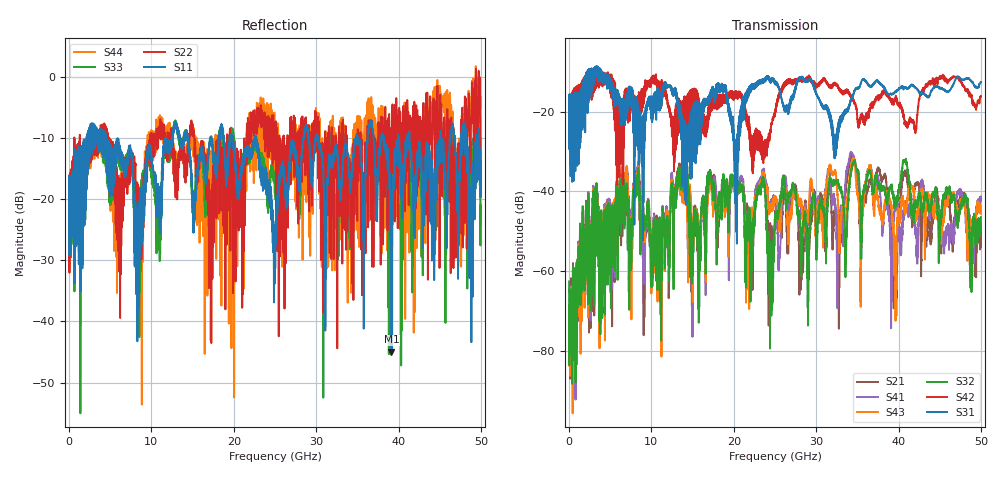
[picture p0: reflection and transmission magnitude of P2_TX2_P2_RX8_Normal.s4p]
!Keysight Technologies,N5225B,MY57041031,A.13.20.10
!Date: Friday, May 31, 2019 11:39:17
!Correction: S11(Full 4 Port(1,2,3,4))
!S12(Full 4 Port(1,2,3,4))
!S13(Full 4 Port(1,2,3,4))
!S14(Full 4 Port(1,2,3,4))
!S21(Full 4 Port(1,2,3,4))
!S22(Full 4 Port(1,2,3,4))
!S23(Full 4 Port(1,2,3,4))
!S24(Full 4 Port(1,2,3,4))
!S31(Full 4 Port(1,2,3,4))
!S32(Full 4 Port(1,2,3,4))
!S33(Full 4 Port(1,2,3,4))
!S34(Full 4 Port(1,2,3,4))
!S41(Full 4 Port(1,2,3,4))
!S42(Full 4 Port(1,2,3,4))
!S43(Full 4 Port(1,2,3,4))
!S44(Full 4 Port(1,2,3,4))
!S4P File: Measurements: <S11,S12,S13,S14>,
!<S21,S22,S23,S24>,
!<S31,S32,S33,S34>,
!<S41,S42,S43,S44>:
# Hz S  dB  R 50.0
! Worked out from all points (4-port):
!   5000 points, 10 MHz to 50 GHz, reference 50 ohm
!   strongest paths, dB at 10 MHz, 12.51 GHz, 25.01 GHz, 37.51 GHz, 50 GHz:
!     S31: -19.4, -14.8, -13.0, -12.4, -12.6
!     S42: -19.7, -21.5, -19.9, -16.3, -16.1
!     S32: -62.5, -39.7, -46.8, -38.3, -46.4
!     S43: -77.9, -38.8, -41.5, -41.8, -45.6
!     S41: -68.5, -37.1, -41.9, -36.2, -41.3
!     S21: -73.2, -37.8, -45.5, -34.1, -54.0
!   lowest |S11| = -44.9 dB at 39.13 GHz (marker M1), VSWR 1.01, Z = 49.6 + j0.422 ohm
!   |S11| at or under -10 dB: 4.481 GHz to 11.72 GHz (7.237 GHz wide, 89.4 % of centre); 22.73 GHz to 28.43 GHz (5.702 GHz wide, 22.3 % of centre); 30.26 GHz to 34.82 GHz (4.558 GHz wide, 14 % of centre)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
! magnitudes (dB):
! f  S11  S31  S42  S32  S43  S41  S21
! 10 MHz  -19.2  -19.4  -19.7  -62.5  -77.9  -68.5  -73.2
! 6.83 GHz  -14.0  -19.5  -19.2  -44.2  -39.3  -40.0  -44.5
! 27.36 GHz  -12.7  -14.7  -12.3  -39.7  -40.7  -40.5  -39.1
! 28.2 GHz  -13.5  -11.4  -12.0  -56.8  -42.5  -45.6  -55.7
! 34.33 GHz  -16.5  -16.7  -16.5  -34.2  -33.0  -30.5  -31.3
! 39.13 GHz  -44.9  -15.7  -17.1  -39.4  -43.4  -58.5  -47.7
! 50 GHz  -14.0  -12.6  -16.1  -46.4  -45.6  -41.3  -54.0
